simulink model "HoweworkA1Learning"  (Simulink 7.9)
settings: Solver=ode45  StartTime=0.0  StopTime=40.0  RelTol=1e-3

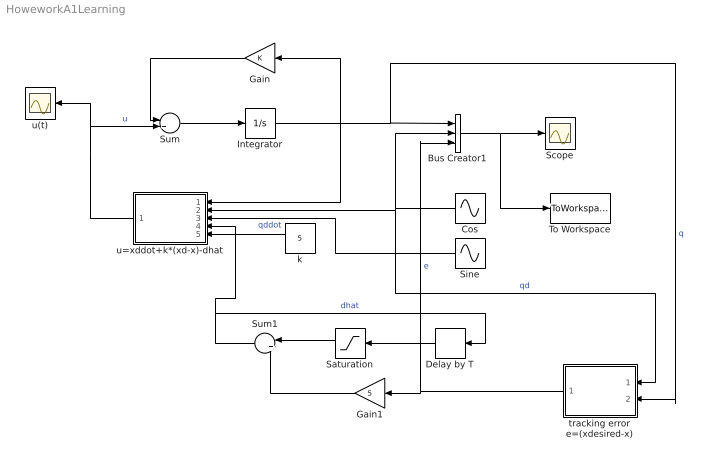
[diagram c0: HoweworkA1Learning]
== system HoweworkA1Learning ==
  Bus Creator1 : BusCreator  Inputs=3
  Cos : Sin  SampleTime=0
  Delay by T : TransportDelay  DelayTime=2*pi
  Gain : Gain
  Gain1 : Gain  Gain=5
  Integrator : Integrator
  Saturation : Saturate  UpperLimit=1  LowerLimit=-1
  Scope : Scope
  Sine : Sin  Phase=pi  SampleTime=0
  Sum : Sum  Inputs=|++
  Sum1 : Sum  Inputs=|+-
  To Workspace : ToWorkspace  VariableName=ICP  SampleTime=-1  SaveFormat=Structure With Time
  k : Constant  Value=5
  tracking error e=(xdesired-x) : MATLAB Function  TreatAsAtomicUnit=on
  u(t) : Scope
  u=xddot+k*(xd-x)-dhat : MATLAB Function  TreatAsAtomicUnit=on
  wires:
  Integrator/1 -> Gain/1, u=xddot+k*(xd-x)-dhat/1(u1), Bus Creator1/1, tracking error e=(xdesired-x)/2(u2)  "q"
  Sum/1 -> Integrator/1
  Gain/1 -> Sum/1
  Bus Creator1/1 -> Scope/1, To Workspace/1
  Cos/1 -> Bus Creator1/2, u=xddot+k*(xd-x)-dhat/2(u2), tracking error e=(xdesired-x)/1(u1)  "qd"
  Saturation/1 -> Sum1/1
  Delay by T/1 -> Saturation/1
  Sum1/1 -> Delay by T/1, u=xddot+k*(xd-x)-dhat/4(u4)  "dhat"
  u=xddot+k*(xd-x)-dhat/1(y) -> Sum/2, u(t)/1  "u"
  Sine/1 -> u=xddot+k*(xd-x)-dhat/3(u3)  "qddot"
  k/1 -> u=xddot+k*(xd-x)-dhat/5(u5)
  tracking error e=(xdesired-x)/1(y) -> Gain1/1, Bus Creator1/3  "e"
  Gain1/1 -> Sum1/2

== matlab function tracking error
e=(xdesired-x) ==
function y = fcn(u1,u2)
%#
xdesired=u1;
x=u2;
e=(xdesired-x);
y=e

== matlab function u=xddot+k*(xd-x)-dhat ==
function y = fcn(u1,u2,u3,u4,u5)
x=u1;
xd=u2;
xddot=u3;
dhat=u4;
k=u3;

u=xddot+k*(xd-x)-dhat;
y=u;
